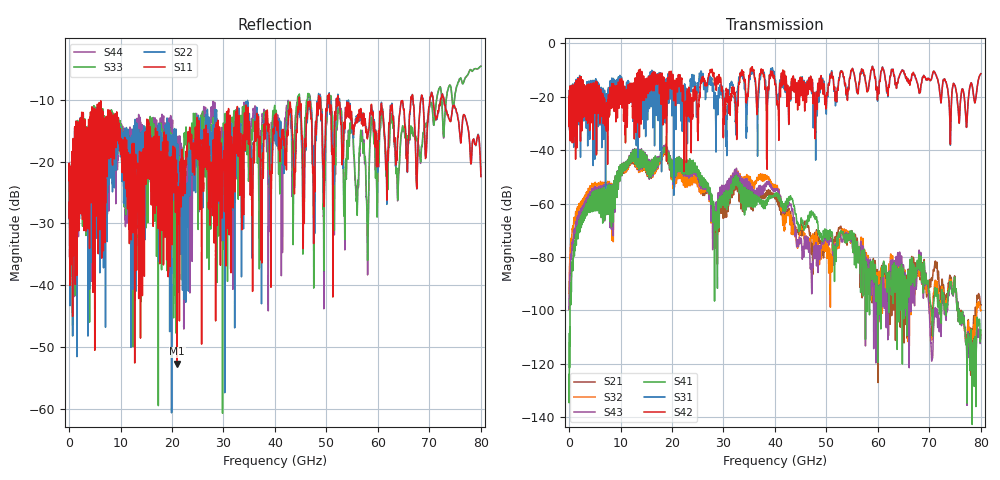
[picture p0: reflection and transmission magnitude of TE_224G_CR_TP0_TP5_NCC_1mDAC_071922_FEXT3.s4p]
!! Reference: tracy_3df_01a_2207
!! CHANNEL DESCRIPTION: TP0_TP5 CR Channel using 1meter DAC, CABLED NCC Host
!! MODEL DESCRIPTION: s4p, FEXT3
!! CONNECTOR DESCRIPTION: OSFP 200G OTB, NCC Socket
!! CABLE DESCRIPTION: 1meter 26AWG Cable
!! MODEL STATUS: Developmental
!! PORT DEFINITIONS:
!! Port  1  ----->  Side A  Side B  <-----  Port  2
!! Port  3  ----->  Side A  Side B  <-----  Port  4
# GHz S MA R 50
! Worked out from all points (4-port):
!   8000 points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, 10 MHz to 80 GHz, reference 50 ohm
!   strongest paths, dB at 10 MHz, 20.01 GHz, 40.01 GHz, 60.01 GHz, 80 GHz:
!     S42: -24.5, -16.2, -15.4, -17.0, -11.4
!     S31: -24.5, -26.1, -13.7, -17.6, -11.4
!     S41: -125.8, -43.7, -56.5, -96.9, -107.4
!     S43: -99.4, -43.8, -55.5, -108.5, -109.1
!     S32: -93.7, -44.6, -54.8, -93.1, -100.0
!     S21: -99.7, -44.4, -58.0, -103.9, -97.9
!   lowest |S11| = -52.7 dB at 21.01 GHz (marker M1), VSWR 1.00, Z = 50 + j0.231 ohm
!   |S11| at or under -10 dB: start of sweep to 44.68 GHz; 52.32 GHz to 66.38 GHz (14.06 GHz wide, 23.7 % of centre); 72.83 GHz to end of sweep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
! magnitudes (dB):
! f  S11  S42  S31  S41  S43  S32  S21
! 10 MHz  -23.1  -24.5  -24.5  -125.8  -99.4  -93.7  -99.7
! 12.36 GHz  -22.4  -25.6  -26.0  -40.1  -39.7  -40.3  -40.7
! 21.01 GHz  -52.7  -17.1  -17.3  -42.7  -42.8  -44.3  -43.8
! 28.53 GHz  -19.4  -15.4  -40.7  -69.6  -63.5  -70.5  -69.5
! 38.78 GHz  -13.9  -17.5  -17.2  -58.0  -52.0  -50.5  -55.5
! 47.15 GHz  -14.0  -15.6  -18.8  -63.5  -93.7  -72.6  -75.5
! 80 GHz  -22.4  -11.4  -11.4  -107.4  -109.1  -100.0  -97.9
